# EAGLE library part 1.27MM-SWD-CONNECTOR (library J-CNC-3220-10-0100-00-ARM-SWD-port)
ARM SWD Programming Header. Example part is the CNC 3220-10-0100-00
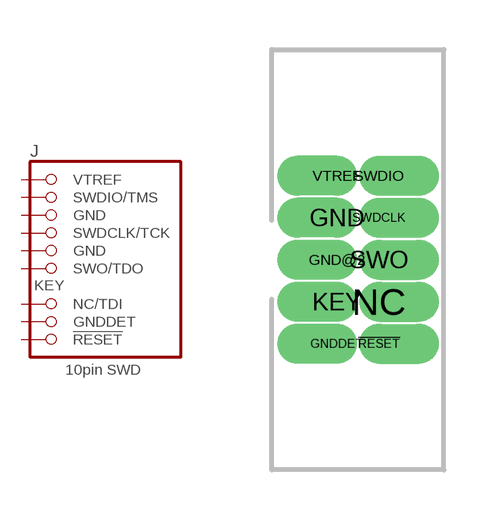
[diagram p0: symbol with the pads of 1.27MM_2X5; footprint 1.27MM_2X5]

Designator prefix J

## 1.27MM-SWD-CONNECTOR  [1.27MM_2X5]
!RESET  !RESET  pas
GND  GND  pas
GND@2  GND  pas
GNDDET  GNDDET  pas
NC  NC/TDI  pas
SWDCLK  SWDCLK/TCK  pas
SWDIO  SWDIO/TMS  pas
SWO  SWO/TDO  pas
VTREF  VTREF  pas

## Footprint 1.27MM_2X5 (pad centres in mm)
drill 0.7 pad 1.016 offset: !RESET 0.635,-2.54; GND -0.635,1.27; GND@2 -0.635,0; GNDDET -0.635,-2.54; KEY -0.635,-1.27; NC 0.635,-1.27; SWDCLK 0.635,1.27; SWDIO 0.635,2.54; SWO 0.635,0; VTREF -0.635,2.54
